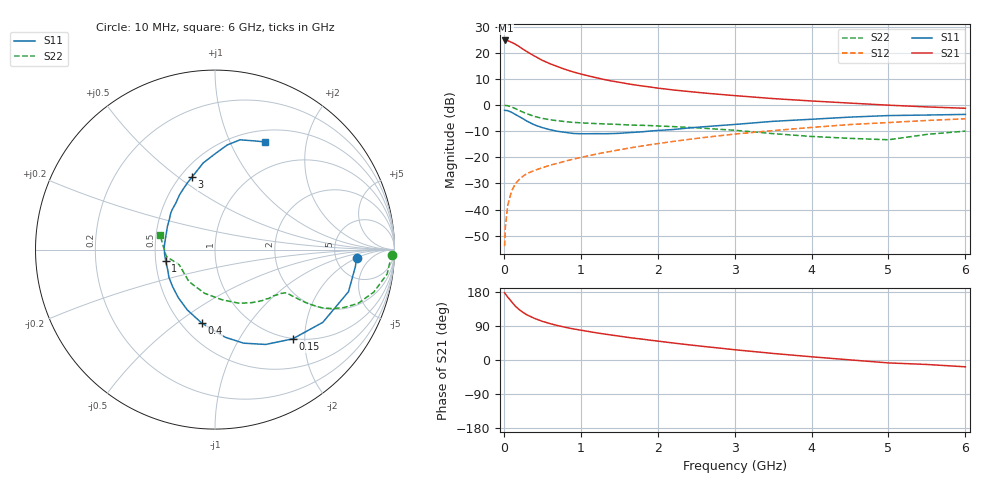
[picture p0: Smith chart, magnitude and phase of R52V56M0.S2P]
! SIEMENS Small Signal Semiconductors
! BFR183
! Si NPN RF Bipolar Junction Transistor in SOT23
! VCE = 2.5 V  IC = 6 mA
! Common Emitter S-Parameters:  May  1996
# GHz  S  MA  R  50
!  f  S11  S21  S12  S22
! GHz  MAG  ANG  MAG  ANG  MAG  ANG  MAG  ANG
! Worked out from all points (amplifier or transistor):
!   36 points, 10 MHz to 6 GHz, reference 50 ohm
!   highest |S21| = 24.7 dB at 20 MHz (marker M1)
!   |S21| within 3 dB of that: start of sweep to 232 MHz
!   unconditionally stable (mu >= 1): 934 MHz to 2.581 GHz
!   at 250 MHz: K = 0.47, MSG = 24.2 dB, |S12| = -27.2 dB
!   at 1.4 GHz: K = 1.06, MAG = 11.9 dB, |S12| = -17.7 dB
!   at 6 GHz: K = 0.89, MSG = 2.0 dB, |S12| = -5.3 dB
!   lowest NFmin = 1.20 dB at 450 MHz
!   S11 on the Smith chart (normalised r, x): 10 MHz: 8.02, -2.06; 150 MHz: 0.99, -1.75; 400 MHz: 0.63, -0.62; 1 GHz: 0.57, -0.08; 3 GHz: 0.57, +0.56; 6 GHz: 0.64, +1.36
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0.01  0.7907 -3.5  16.97 177.4  0.002 88.7  0.9874 -1.6
0.02  0.7878 -6.9  17.12 174.3  0.0047 84.4  0.9797 -3.2
0.05  0.7799 -17.5  16.97 166.2  0.012 81.9  0.9685 -8.1
0.1  0.7247 -34.0  15.77 153.9  0.0225 72.7  0.9156 -15.0
0.15  0.6592 -49.0  14.48 142.0  0.0313 67.1  0.8518 -20.6
0.2  0.5991 -61.9  13.05 133.0  0.0376 63.5  0.7859 -24.3
0.25  0.5451 -73.0  11.62 125.5  0.0437 60.4  0.7287 -26.8
0.3  0.4914 -83.4  10.46 119.1  0.0488 59.2  0.6811 -28.5
0.4  0.4155 -100.4  8.591 109.7  0.0563 57.3  0.6036 -30.1
0.5  0.3695 -114.8  7.138 102.1  0.0632 57.4  0.5537 -30.6
0.6  0.3369 -127.4  6.151 96.1  0.0704 57.4  0.5223 -30.8
0.8  0.2997 -148.9  4.778 86.3  0.0845 58.6  0.4806 -31.1
1  0.2818 -166.9  3.906 78.7  0.0992 59.9  0.4561 -31.9
1.1  0.282 -174.6  3.596 75.3  0.1071 60.3  0.4482 -32.9
1.3  0.2822 171.9  3.078 68.8  0.1231 60.3  0.435 -34.5
1.6  0.2944 154.3  2.555 60.0  0.1474 59.8  0.4169 -38.0
2.2  0.3396 129.8  1.939 44.9  0.2009 57.2  0.3864 -47.4
3  0.4243 107.5  1.511 27.1  0.2778 50.1  0.3287 -65.5
3.5  0.487 97.8  1.325 17.3  0.3239 44.3  0.2834 -81.6
4.5  0.5864 83.4  1.086 0.3  0.4229 32.3  0.2301 -129.2
5.5  0.6422 70.7  0.918 -11.8  0.5057 19.9  0.2743 -172.1
6  0.6608 65.3  0.865 -18.0  0.5443 11.8  0.3165 165.2
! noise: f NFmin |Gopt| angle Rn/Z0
0.45  1.2  0.21  41  0.24
0.9  1.25  0.24  101  0.21
1.8  2  0.32  175  0.14
